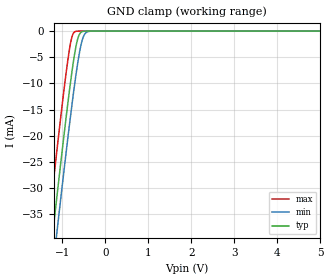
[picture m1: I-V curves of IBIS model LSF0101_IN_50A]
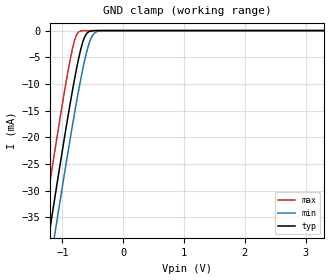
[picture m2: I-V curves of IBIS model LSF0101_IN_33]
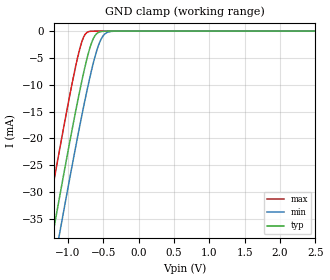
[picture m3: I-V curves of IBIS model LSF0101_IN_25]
|Texas Instruments Incorporated
| Single Bidirectional Multi-Voltage Level Translator
| for Open-Drain & Push-Pull Application
| Marketing part#   Digital Voltage Range   Package-type   #pins
| LSF0101   1.2V-5.5V   QFN   6
| This device can be powered at the following Vccs:
|  5 volt Vcc
|  3.3 volt Vcc
|  2.5 volt Vcc
|  1.8 volt Vcc
|  1.2 volt Vcc
[IBIS Ver]   4.1
[File name]   lsf0101.ibs
[File Rev]   1.0
[Date]   12/18/2013
[Source]
| Texas Instruments Incorporated.
| 12500 TI Blvd
| Dallas, TX -75243
[Notes]   Revision History:
| Rev 1.0: 12/18/2013
| - Initial version of the model
| - Model generated from simulations in TISPICE
| - C_comp although listed in numerical order of value are
|   obtained from varying PVT conditions. For PVT conditions for
|   each specific value refer the buffer description under
|   respective [Model]. IBIS model user is responsible for using
|   appropriate C_comp to simulate for Signal Integrity.
| - Non-monotonic data due to FET characteristics.
| - POWER clamp data deleted as there is no power-clmp diode.
[Disclaimer]
| This model is designed as an aid for customers of Texas Instruments.
| TI and its licensors and suppliers make no warranties, either expressed
| or implied, with respect to this  model, including the warranties of
| merchantability or fitness for a particular purpose. The model is
| provided solely on an "as is" basis. The entire risk as to its quality
| and performance is with the customer.
| This file provides unique models under the [Model Selector] for each Vcc.
| For operation at a specific Vcc, select the appropriate model after each
| [Model Selector] keyword.
[Copyright]
 (C) Copyright 2013 Texas Instruments Incorporated.All rights reserved.
|   Device
[Component]   LSF0101
[Manufacturer]   TI
[Package]
|   typ   min   max
R_pkg   0.0521   0.0464   0.0562
L_pkg   0.4298nH   0.3766nH   0.4721nH
C_pkg   0.1097pF   0.1074pF   0.1120pF
[Pin]  signal_name   model_name   R_pin   L_pin   C_pin
1   GND   GND   0.05616   0.47211nH   0.11202pF
2   VREF_A   LSF0101_IO   0.04639   0.37661nH   0.10736pF
3   A1   LSF0101_IO   0.05393   0.44988nH   0.10979pF
4   B1   LSF0101_IO   0.05422   0.4482nH   0.10984pF
5   VREF_B   LSF0101_IO   0.04709   0.37684nH   0.10786pF
6   EN   LSF0101_IN   0.05494   0.45541nH   0.11112pF
[Series Switch Groups]
| Function Group States
On  1 /   | A1 -> B1 EN HIGH
Off 1 /   | EN LOW
[Series Pin Mapping]   pin_2   model_name   function_table_group
3   4   LSF0101_IO_S   1
| Model LSF0101_IN
[Model Selector]   LSF0101_IN
LSF0101_IN_50A   5 volt Vcc
LSF0101_IN_33   3.3 volt Vcc
LSF0101_IN_25   2.5 volt Vcc
LSF0101_IN_18   1.8 volt Vcc
LSF0101_IN_12A   1.2 volt Vcc
| Model LSF0101_IO
[Model Selector]   LSF0101_IO
LSF0101_IO_50A   5 volt Vcc
LSF0101_IO_33   3.3 volt Vcc
LSF0101_IO_25   2.5 volt Vcc
LSF0101_IO_18   1.8 volt Vcc
LSF0101_IO_12A   1.2 volt Vcc
| Model LSF0101_IO_S
[Model Selector]   LSF0101_IO_S
LSF0101_IO_50A_S   5 volt Vcc
LSF0101_IO_33_S   3.3 volt Vcc
LSF0101_IO_25_S   2.5 volt Vcc
LSF0101_IO_18_S   1.8 volt Vcc
LSF0101_IO_12A_S   1.2 volt Vcc
[Model]   LSF0101_IO_50A_S
Model_type  Series_switch
| variable   typ   min   max
C_comp   0   0   0
[Temperature Range]   40   100   -40
| Ambient temperature   25   85   -40
[Voltage range]   5   5   5
[On]
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[Off]
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[Model]   LSF0101_IO_33_S
Model_type  Series_switch
| variable   typ   min   max
C_comp   0   0   0
[Temperature Range]   40   100   -40
| Ambient temperature   25   85   -40
[Voltage range]   3.3   3   3.6
[On]
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[Off]
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[Model]   LSF0101_IO_25_S
Model_type  Series_switch
| variable   typ   min   max
C_comp   0   0   0
[Temperature Range]   40   100   -40
| Ambient temperature   25   85   -40
[Voltage range]   2.5   2.3   2.7
[On]
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[Off]
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[Model]   LSF0101_IO_18_S
Model_type  Series_switch
| variable   typ   min   max
C_comp   0   0   0
[Temperature Range]   40   100   -40
| Ambient temperature   25   85   -40
[Voltage range]   1.8   1.65   1.95
[On]
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[Off]
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[Model]   LSF0101_IO_12A_S
Model_type  Series_switch
| variable   typ   min   max
C_comp   0   0   0
[Temperature Range]   40   100   -40
| Ambient temperature   25   85   -40
[Voltage range]   1.2   1.2   1.2
[On]
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[Off]
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| Models and submodels in the file (15): LSF0101_IN_50A (Input), LSF0101_IN_33 (Input), LSF0101_IN_25 (Input), LSF0101_IN_18 (Input), LSF0101_IN_12A (Input), LSF0101_IO_50A_S (Series_switch), LSF0101_IO_50A (Terminator), LSF0101_IO_33_S (Series_switch), LSF0101_IO_33 (Terminator), LSF0101_IO_25_S (Series_switch), LSF0101_IO_25 (Terminator), LSF0101_IO_18_S (Series_switch), LSF0101_IO_18 (Terminator), LSF0101_IO_12A_S (Series_switch), LSF0101_IO_12A (Terminator)
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[Model]   LSF0101_IN_50A
Model_type  Input
Vinl=0.6
Vinh=5
| variable   typ   min   max
C_comp   6.26pF   4.66pF   9.23pF
[Temperature Range]   40   100   -40
| Ambient temperature   25   85   -40
[Voltage range]   5   5   5
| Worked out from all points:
|   GND clamp passes 1 mA (typ) near -0.62 V on its own axis
[GND Clamp]
| PCA9306_IN_50A
|   Voltage   I(typ)   I(min)   I(max)
-5V       -328.9mA   -335.1mA   -321mA
-1.365V   -49.02mA   -55.82mA   -40.25mA
-1.325V   -46.04mA   -52.85mA   -37.26mA
-1.215V   -37.92mA   -44.74mA   -29.12mA
-1.12V    -30.99mA   -37.81mA   -22.19mA
-850mV    -12.22mA   -18.79mA   -4.2mA
-780mV    -7.858mA   -14.16mA   -1.166mA
-710mV    -4.062mA   -9.799mA   -118uA
-635mV    -1.238mA   -5.618mA   -5.709uA
-555mV    -167.5uA   -2.206mA   -200.7nA
-405mV    -1.746uA   -97.01uA   -397.3pA
5V        97.63pA    2.873nA    90.01pA
[Model]   LSF0101_IN_33
Model_type  Input
Vinl=0.6
Vinh=3.6
| variable   typ   min   max
C_comp   6.06pF   4.74pF   7.90pF
[Temperature Range]   40   100   -40
| Ambient temperature   25   85   -40
[Voltage range]   3.3   3   3.6
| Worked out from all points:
|   GND clamp passes 1 mA (typ) near -0.62 V on its own axis
[GND Clamp]
| PCA9306_IN_33
|   Voltage   I(typ)   I(min)   I(max)
-3.3V     -197mA     -203.5mA   -188.9mA
-1.36V    -48.65mA   -55.45mA   -39.88mA
-1.315V   -45.3mA    -52.12mA   -36.52mA
-1.23V    -39.02mA   -45.85mA   -30.22mA
-1.19V    -36.09mA   -42.91mA   -27.28mA
-1.115V   -30.63mA   -37.45mA   -21.83mA
-850mV    -12.22mA   -18.79mA   -4.2mA
-715mV    -4.305mA   -10.1mA    -142.6uA
-635mV    -1.238mA   -5.618mA   -5.709uA
-555mV    -167.5uA   -2.206mA   -200.7nA
-405mV    -1.746uA   -97.01uA   -397.3pA
3.3V      64.05pA    2.84nA     56.56pA
[Model]   LSF0101_IN_25
Model_type  Input
Vinl=0.6
Vinh=2.7
| variable   typ   min   max
C_comp   5.97pF   4.76pF   7.97pF
[Temperature Range]   40   100   -40
| Ambient temperature   25   85   -40
[Voltage range]   2.5   2.3   2.7
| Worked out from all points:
|   GND clamp passes 1 mA (typ) near -0.62 V on its own axis
[GND Clamp]
| PCA9306_IN_25
|   Voltage   I(typ)   I(min)   I(max)
-2.5V     -135.3mA   -141.9mA   -127mA
-1.335V   -46.79mA   -53.6mA    -38.01mA
-1.22V    -38.29mA   -45.11mA   -29.48mA
-1.185V   -35.72mA   -42.55mA   -26.92mA
-1.12V    -30.99mA   -37.81mA   -22.19mA
-855mV    -12.54mA   -19.12mA   -4.472mA
-785mV    -8.155mA   -14.49mA   -1.319mA
-720mV    -4.553mA   -10.4mA    -171.8uA
-640mV    -1.37mA    -5.873mA   -7.034uA
-560mV    -192.8uA   -2.373mA   -247.3nA
-415mV    -2.384uA   -124.1uA   -599.6pA
2.5V      48.96pA    2.825nA    41.29pA
